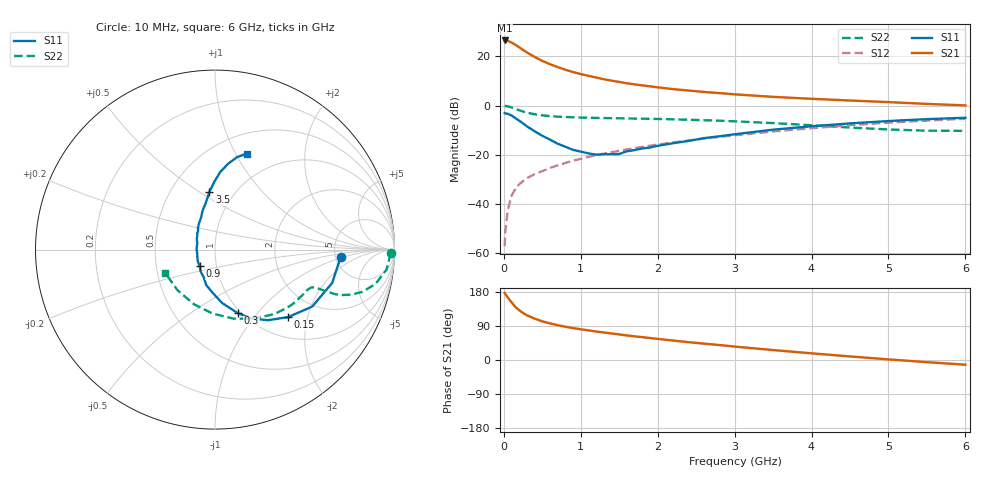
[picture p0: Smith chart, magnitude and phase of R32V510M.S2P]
! SIEMENS Small Signal Semiconductors
! BFR181
! Si NPN RF Bipolar Junction Transistor in SOT23
! VCE = 2.5 V  IC = 10 mA
! Common Emitter S-Parameters:  May  1996
# GHz  S  MA  R  50
!  f  S11  S21  S12  S22
! GHz  MAG  ANG  MAG  ANG  MAG  ANG  MAG  ANG
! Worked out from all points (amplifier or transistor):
!   36 points, 10 MHz to 6 GHz, reference 50 ohm
!   highest |S21| = 26.4 dB at 10 MHz (marker M1)
!   |S21| within 3 dB of that: start of sweep to 210.1 MHz
!   unconditionally stable (mu >= 1): 698.5 MHz to 2.65 GHz
!   at 250 MHz: K = 0.62, MSG = 26.6 dB, |S12| = -30.7 dB
!   at 1.4 GHz: K = 1.08, MAG = 12.8 dB, |S12| = -19.0 dB
!   at 6 GHz: K = 0.85, MSG = 2.7 dB, |S12| = -5.4 dB
!   S11 on the Smith chart (normalised r, x): 10 MHz: 5.56, -0.91; 150 MHz: 1.40, -1.52; 300 MHz: 0.97, -0.80; 900 MHz: 0.83, -0.16; 3.5 GHz: 0.77, +0.55; 6 GHz: 0.71, +1.11
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0.01  0.702 -3.4  20.88 176.8  0.0014 86.0  0.9809 -1.2
0.02  0.6924 -6.5  20.84 173.7  0.0028 83.3  0.9741 -2.6
0.05  0.6788 -15.9  20.51 165.3  0.0074 82.6  0.9623 -6.6
0.1  0.6277 -30.4  18.95 152.2  0.0148 78.3  0.9144 -12.1
0.15  0.5537 -42.8  17.07 140.0  0.0204 71.6  0.854 -16.0
0.2  0.4916 -53.2  15.15 131.3  0.0253 69.3  0.7991 -18.3
0.25  0.4338 -62.1  13.39 124.0  0.0293 68.2  0.7547 -19.6
0.3  0.3775 -70.1  11.93 117.9  0.0336 67.2  0.7173 -20.3
0.4  0.3004 -82.4  9.678 109.3  0.0404 68.0  0.6639 -20.6
0.5  0.2424 -92.8  8.034 102.0  0.0466 68.2  0.6308 -20.6
0.6  0.2031 -104.0  6.884 96.6  0.054 68.9  0.6091 -20.7
0.7  0.1675 -111.8  6.02 91.9  0.0609 69.6  0.5938 -20.9
0.9  0.1257 -132.7  4.763 84.2  0.0758 69.8  0.5761 -21.5
1.1  0.1068 -157.0  3.998 78.2  0.0903 70.2  0.5652 -23.0
1.3  0.1027 -179.6  3.412 72.6  0.1058 69.8  0.5569 -24.8
1.6  0.1179 149.7  2.826 64.7  0.129 69.0  0.5475 -28.1
2.2  0.1719 121.2  2.149 51.3  0.1782 66.0  0.5246 -36.2
3  0.2608 101.7  1.686 35.4  0.2488 60.0  0.4776 -49.8
3.5  0.3237 95.5  1.497 26.2  0.2967 55.4  0.4395 -61.1
4.5  0.4336 86.1  1.262 9.4  0.3977 44.2  0.357 -91.9
5.5  0.5292 76.6  1.077 -5.7  0.4946 30.9  0.308 -132.7
6  0.5639 71.7  1.005 -12.4  0.5378 23.6  0.3061 -154.8
